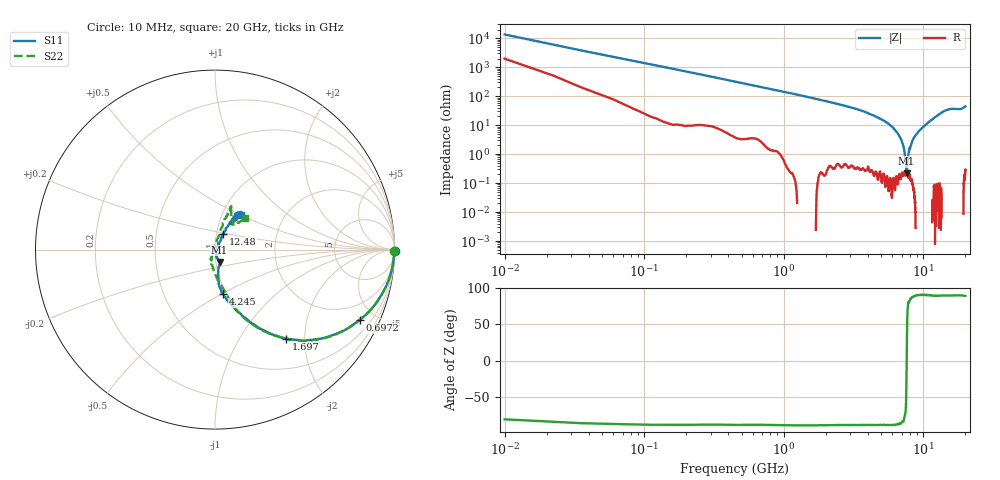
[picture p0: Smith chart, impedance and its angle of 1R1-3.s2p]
!Keysight Technologies,P5008B,MY61100088,A.16.20.02
!Date: Monday, May 27, 2024 13:54:33
!Correction: S11(C  2-Port  )
!S21(C  2-Port  )
!S12(C  2-Port  )
!S22(C  2-Port  )
!S2P File: Measurements: S11, S21, S12, S22:
# Hz S  dB  R 50
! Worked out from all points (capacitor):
!   1601 points, 10 MHz to 20 GHz, reference 50 ohm
!   read as one part in series: C = 1.12 pF near 110 MHz
!   lowest |Z| = 215 mohm at 7.581 GHz (marker M1)
!   series resonance near 7.586 GHz, so ESL is about 390 pH
!   S11 on the Smith chart (normalised r, x): 10 MHz: open; 697.2 MHz: 1.03, -4.09; 1.697 GHz: 0.98, -1.62; 4.245 GHz: 0.96, -0.51; 12.48 GHz: 1.08, +0.19; 20 GHz: 1.22, +0.50
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1e7  0.01 -0.4  -42.63 81.2  -42.62 81.3  -0.02 -0.4
1.349375e8  -0.06 -5.5  -20.46 83.7  -20.47 83.8  -0.05 -5.6
2.223938e8  -0.13 -9.0  -16.32 80.1  -16.33 80.2  -0.13 -9.0
4.098e8  -0.39 -16.1  -11.20 73.1  -11.21 73.1  -0.38 -16.3
6.971562e8  -0.96 -25.9  -7.23 63.2  -7.24 63.2  -0.96 -26.3
1.696656e9  -3.95 -51.5  -2.23 38.5  -2.24 38.5  -3.92 -51.4
3.345831e9  -9.02 -71.0  -0.57 18.2  -0.58 18.2  -9.12 -70.8
4.245381e9  -11.92 -79.6  -0.29 11.3  -0.30 11.3  -12.11 -75.9
6.681662e9  -19.74 -78.2  -0.02 -0.7  -0.03 -0.7  -19.87 -96.6
7.581212e9  -22.63 -69.6  0.00 -3.8  -0.00 -3.8  -23.32 -108.1
9.017994e9  -26.07 -76.3  0.03 -8.4  0.02 -8.5  -26.98 -115.2
1.0005e10  -32.99 -75.9  0.05 -11.4  0.03 -11.3  -34.01 -118.2
1.041729e10  -39.00 -51.6  0.05 -12.5  0.04 -12.5  -39.62 -143.8
1.065468e10  -37.59 4.3  0.05 -13.2  0.03 -13.2  -43.42 145.9
1.134183e10  -28.25 63.2  0.04 -15.3  0.04 -15.2  -29.37 77.3
1.195402e10  -22.79 62.5  0.02 -16.9  0.02 -16.9  -23.40 74.8
1.247876e10  -20.10 62.0  0.01 -18.4  0.00 -18.4  -20.22 73.2
1.334083e10  -15.94 61.1  -0.05 -20.9  -0.06 -20.8  -15.99 72.9
1.476512e10  -12.47 59.5  -0.18 -24.9  -0.19 -24.8  -12.44 68.7
1.667666e10  -12.62 53.8  -0.17 -28.5  -0.17 -28.5  -12.55 67.4
1.841329e10  -15.46 57.6  -0.05 -32.9  -0.06 -32.9  -15.22 54.7
2e10  -12.43 53.1  -0.21 -38.4  -0.22 -38.4  -12.28 46.2
